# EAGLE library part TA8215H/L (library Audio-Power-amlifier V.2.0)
Toshiba 18W BTLx2CH AUDIO POWER AMPLIFIER
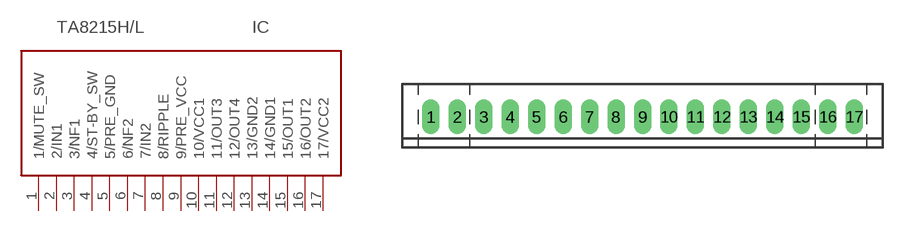
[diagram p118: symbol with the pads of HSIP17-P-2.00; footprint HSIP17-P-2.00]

Designator prefix IC

## TA8215H/LTA8215H  [HSIP17-P-2.00]
1  1/MUTE_SW
2  2/IN1  in
3  3/NF1  in
4  4/ST-BY_SW
5  5/PRE_GND  pwr
6  6/NF2  in
7  7/IN2  in
8  8/RIPPLE
9  9/PRE_VCC
10  10/VCC1  pwr
11  11/OUT3  out
12  12/OUT4  out
13  13/GND2  pwr
14  14/GND1  pwr
15  15/OUT1  out
16  16/OUT2  out
17  17/VCC2  pwr

## TA8215H/LTA8215L  [HSIP17-P-2.00]
Pads as for HSIP17-P-2.00

## Footprint HSIP17-P-2.00 (pad centres in mm)
HSIP17-P-2.00 Source: http://www.semicon.toshiba.co.jp/td/en/ASSP/Audio_ICs/en_20050517_TA8210ALQ_datasheet.pdf
drill 0.8 pad 1.2 long: 1 -16,0; 2 -14,0; 3 -12,0; 4 -10,0; 5 -8,0; 6 -6,0; 7 -4,0; 8 -2,0; 9 0,0; 10 2,0; 11 4,0; 12 6,0; 13 8,0; 14 10,0; 15 12,0; 16 14,0; 17 16,0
